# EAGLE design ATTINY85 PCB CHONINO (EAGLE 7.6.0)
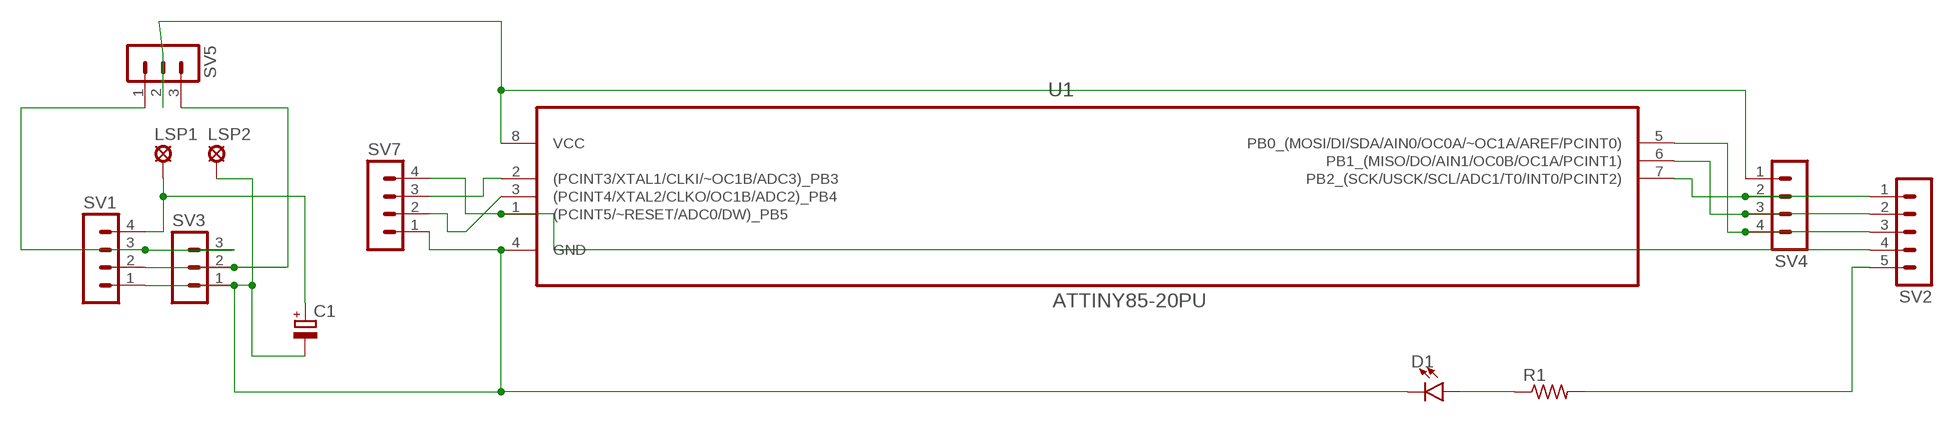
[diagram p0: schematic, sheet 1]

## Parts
C1  CPOL-EUE3.5-8  [E3,5-8]
D1  LED3MM  [LED_3MM]
LSP1  LSP11  [LSP11]
LSP2  LSP11  [LSP11]
R1  R-US_0207/10  [0207/10]
SV1  MA04-1  [MA04-1]
SV2  MA05-1  [MA05-1]
SV3  MA03-1  [MA03-1]
SV4  MA04-1  [MA04-1]
SV5  MA03-1  [MA03-1]
SV7  MA04-1  [MA04-1]
U1  ATTINY85-20PU  [DIP254P762X533-8]

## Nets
N$1: SV2.4 SV7.4 U1.1((PCINT5/~RESET/ADC0/DW)_PB5)
N$2: SV7.3 U1.2((PCINT3/XTAL1/CLKI/~OC1B/ADC3)_PB3)
N$3: SV7.2 U1.3((PCINT4/XTAL2/CLKO/OC1B/ADC2)_PB4)
N$4: SV2.3 SV4.4 U1.5(PB0_(MOSI/DI/SDA/AIN0/OC0A/~OC1A/AREF/PCINT0))
N$6: SV2.1 SV4.2 U1.7(PB2_(SCK/USCK/SCL/ADC1/T0/INT0/PCINT2))
N$7: SV2.2 SV4.3 U1.6(PB1_(MISO/DO/AIN1/OC0B/OC1A/PCINT1))
N$8: SV4.1 SV5.2 U1.8(VCC)
N$9: D1.A R1.1
N$10: R1.2 SV2.5
N$11: C1.- D1.K(C) LSP2.MP SV1.1 SV3.1 SV7.1 U1.4(GND)
N$12: SV1.2 SV3.2 SV5.3
N$13: SV1.3 SV3.3 SV5.1
N$16: C1.+ LSP1.MP SV1.4

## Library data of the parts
C1 = resistor:CPOL-EU: POLARIZED CAPACITOR, European symbol
D1 = SparkFun-LED:LED: LED (Generic); PROD_ID: DIO-08794
LSP1 LSP2 = solpad:LSP11: SOLDER PAD
R1 = rcl:R-US_: RESISTOR, American symbol
SV1 SV4 SV7 = con-lstb:MA04-1: PIN HEADER; OC_FARNELL: unknown; OC_NEWARK: unknown
SV2 = con-lstb:MA05-1: PIN HEADER; OC_FARNELL: unknown; OC_NEWARK: unknown
SV3 SV5 = con-lstb:MA03-1: PIN HEADER; OC_FARNELL: unknown; OC_NEWARK: unknown
U1 = Atmel_By_element14_Batch_1-00:ATTINY85-20PU: 8-bit Microcontroller with In-System Programmable Flash; MPN: ATTINY85-20PU; OC_FARNELL: 1455162; OC_NEWARK: 58M3796; PACKAGE: PDIP-8; SUPPLIER: Atmel

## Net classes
0 default: clearance 0.205 mm

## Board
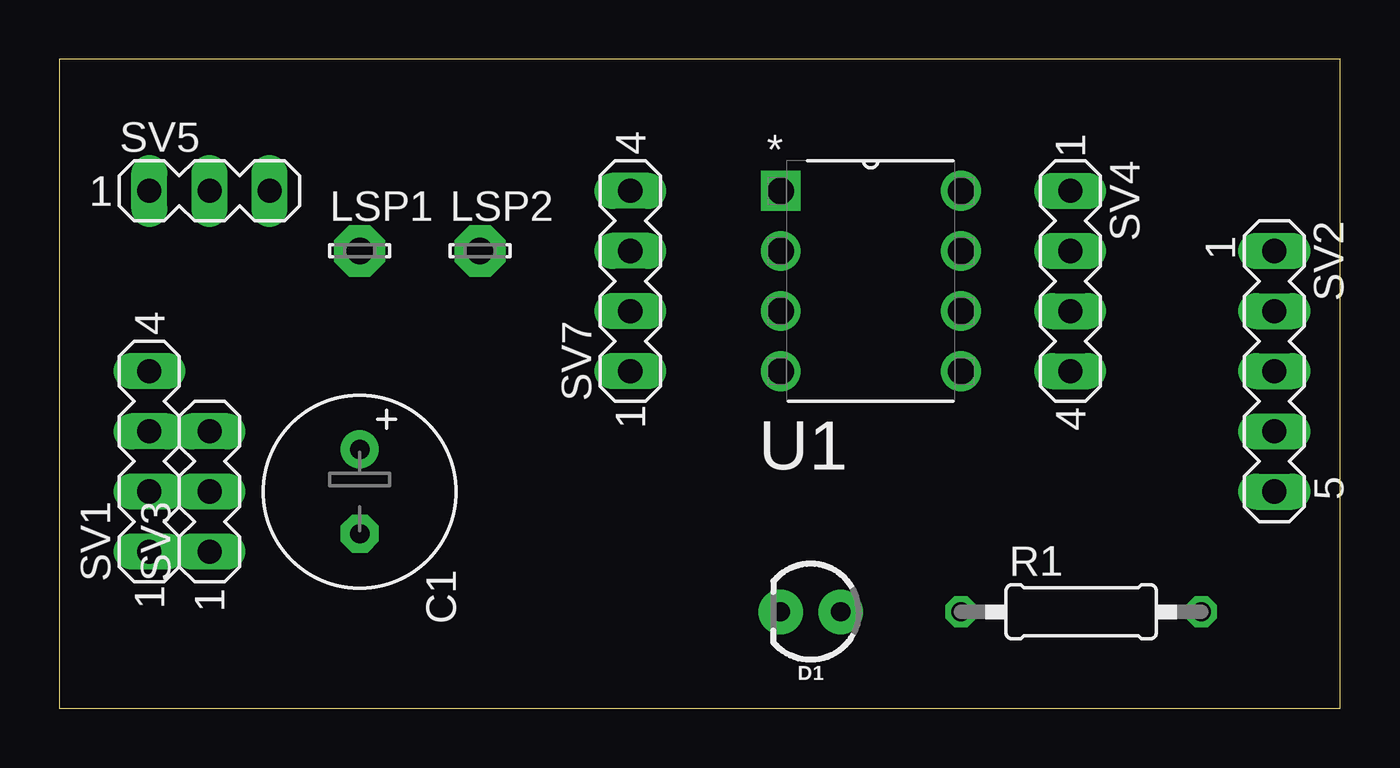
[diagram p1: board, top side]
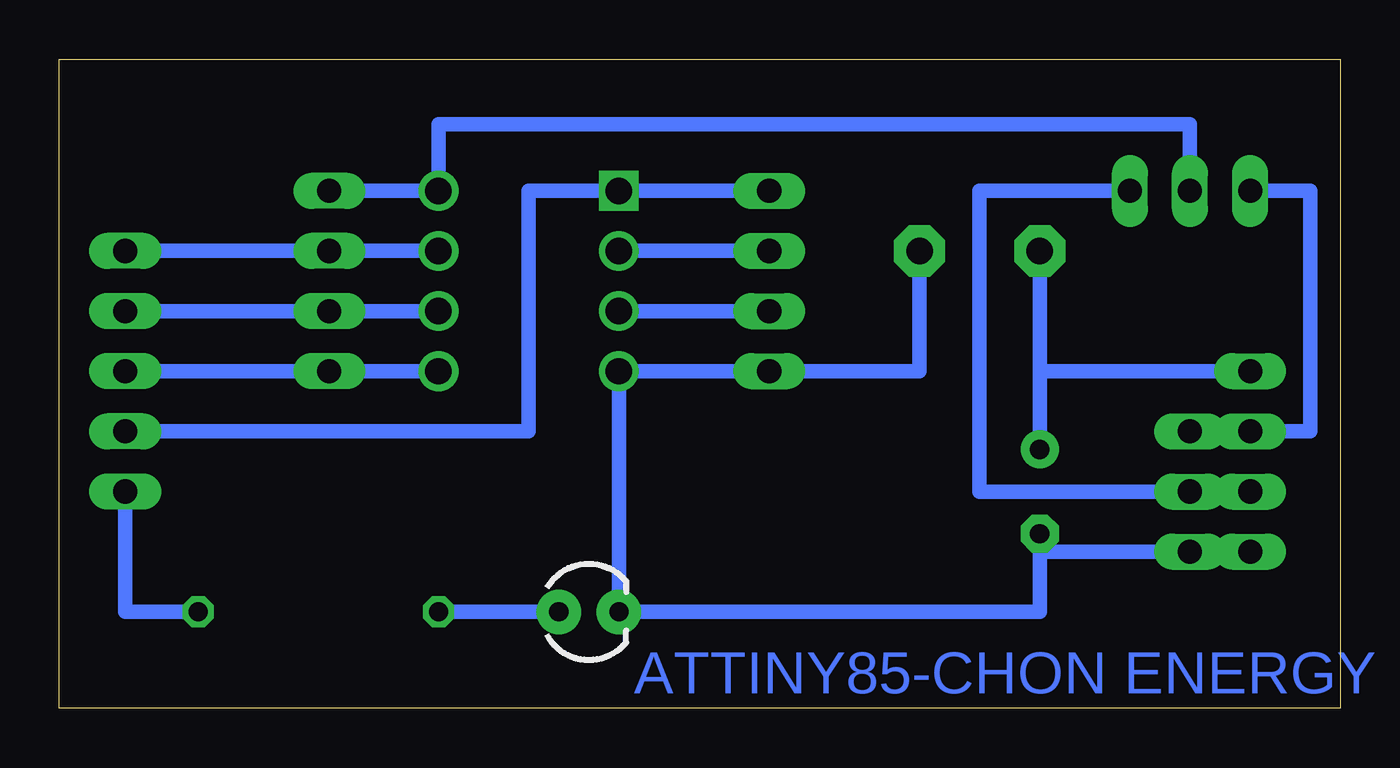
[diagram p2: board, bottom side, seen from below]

Size 54.13 x 27.42 mm. Coordinates in mm from the lower left corner, seen from the top.
Outline: 0,0 54.13,0 54.13,27.42 0,27.42 0,0
Copper layers (1*16): Top 0.035mm / dielectric 1.5mm / Bottom 0.035mm
Design rules "default": minimum track width 10mil, minimum drill 24mil, track to track 8mil, track to pad 8mil, pad to pad 8mil, via to via 8mil, smd to smd 8mil, copper to edge 40mil, drill to drill 8mil, minimum pad ring 10mil, minimum via ring 8mil, stop-mask expansion 4mil, vias tented up to drill 0mil, thermal gap 10mil

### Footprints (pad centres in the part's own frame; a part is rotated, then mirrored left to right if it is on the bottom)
E3,5-8 = drill 0.813 pad 1.6: + -1.778,0 | drill 0.813 pad 1.6 octagon: - 1.778,0
LED_3MM = drill 0.813 pad 1.88: A -1.27,0; K 1.27,0
LSP11 = drill 1.118 pad 2.159 octagon: MP 0,0
0207/10 = drill 0.813 octagon: 1 -5.08,0; 2 5.08,0
MA04-1 = drill 1.016 long: 1 -3.81,0; 2 -1.27,0; 3 1.27,0; 4 3.81,0
MA05-1 = drill 1.016 long: 1 -5.08,0; 2 -2.54,0; 3 0,0; 4 2.54,0; 5 5.08,0
MA03-1 = drill 1.016 long: 1 -2.54,0; 2 0,0; 3 2.54,0
DIP254P762X533-8 = drill 1.118 square: 1 -7.62,7.62 | drill 1.118: 2 -7.62,5.08; 3 -7.62,2.54; 4 -7.62,0; 5 0,0; 6 0,2.54; 7 0,5.08; 8 0,7.62

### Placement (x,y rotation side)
C1  12.7,9.16 270 top
D1  31.75,4.08 180 top
LSP1  12.7,19.32 0 top
LSP2  17.78,19.32 0 top
R1  43.18,4.08 0 top
SV1  3.81,10.43 90 top
SV2  51.34,14.24 270 top
SV3  6.35,9.16 90 top
SV4  42.72,18.05 270 top
SV5  6.35,21.86 0 top
SV7  24.13,18.05 90 top
U1  38.1,14.24 0 top

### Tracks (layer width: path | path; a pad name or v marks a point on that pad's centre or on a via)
N$1
  Bottom 0.61: SV7.4 U1.1 34.29,21.86 34.29,11.7 SV2.4
N$2
  Bottom 0.61: SV7.3 U1.2
N$3
  Bottom 0.61: SV7.2 U1.3
N$4
  Bottom 0.61: U1.5 SV4.4 SV2.3
N$6
  Bottom 0.61: U1.7 SV4.2 SV2.1
N$7
  Bottom 0.61: U1.6 SV4.3 SV2.2
N$8
  Bottom 0.61: SV4.1 U1.8 38.1,24.67 6.35,24.67 SV5.2
N$9
  Bottom 0.61: R1.1 D1.A
N$10
  Bottom 0.61: R1.2 51.34,4.08 SV2.5
N$11
  Bottom 0.61: SV1.1 SV3.1 12.7,6.62 C1.- 12.7,4.08 D1.K U1.4 SV7.1 17.78,14.24 LSP2.MP
N$12
  Bottom 0.61: SV1.2 SV3.2 15.24,9.16 15.24,21.86 SV5.3
N$13
  Bottom 0.61: SV3.3 SV1.3 1.27,11.7 1.27,21.86 SV5.1
N$16
  Bottom 0.61: SV1.4 12.7,14.24 | 12.7,14.24 LSP1.MP | C1.+ 12.7,14.24

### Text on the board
Bottom: ATTINY85-CHON ENERGY

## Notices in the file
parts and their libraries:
SparkFun-LED: Licensing: Creative Commons ShareAlike 4.0 International - https://creativecommons.org/licenses/by-sa/4.0
